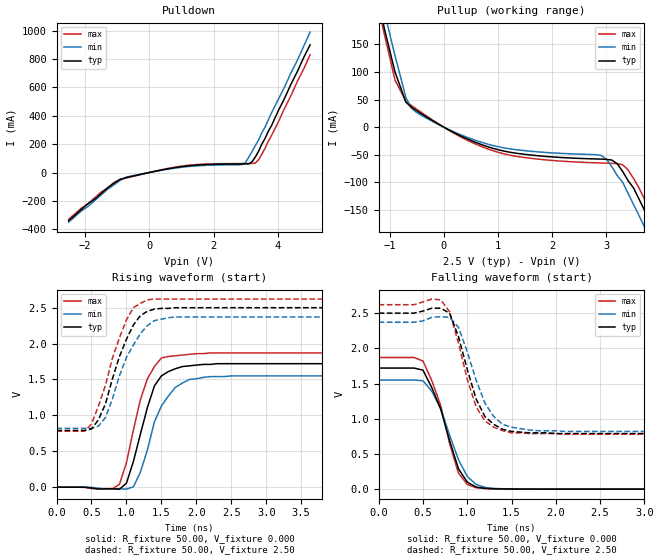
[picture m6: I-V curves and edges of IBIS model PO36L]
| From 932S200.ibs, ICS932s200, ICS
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|   Model PO36L
[Model]   PO36L
Model_type   Output
Polarity   Non-Inverting
Vmeas =   1.25V
Cref =  20.00pF
Rref =  0.000
Vref =   1.25V
C_comp   5.50pF   5.00pF   6.00pF
[Temperature Range]   27.00   70.00   0.000
[Voltage Range]   2.50V   2.37V   2.62V
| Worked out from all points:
|   slope of the pulldown table from 0 to 0.375 V, typ, clamps not added: 21.3 ohm
|   slope of the pullup table from 0 to 0.375 V, typ, clamps not added: 20 ohm
|   rising waveform, R_fixture 50.00, V_fixture 0.000: 20-80 % time 294ps typ, 346ps min, 288ps max; typ from 0 V to 1.72 V
|   rising waveform, R_fixture 50.00, V_fixture 2.50: 20-80 % time 362ps typ, 388ps min, 363ps max; typ from 0.79 V to 2.5 V
|   falling waveform, R_fixture 50.00, V_fixture 0.000: 20-80 % time 265ps typ, 286ps min, 253ps max; typ from 1.72 V to 0 V
|   falling waveform, R_fixture 50.00, V_fixture 2.50: 20-80 % time 257ps typ, 279ps min, 250ps max; typ from 2.5 V to 0.79 V
[Pulldown]
| voltage   I(typ)   I(min)   I(max)
-2.5V     -340mA     -350mA     -330mA
-1.1V     -77.43mA   -88.38mA   -71.31mA
-900mV    -48.05mA   -55.1mA    -48.31mA
-700mV    -34.95mA   -32mA      -37.73mA
1.2V      46.86mA    41.63mA    50.55mA
2.8V      59.88mA    54.77mA    63.39mA
3V        60.16mA    72.42mA    63.65mA
3.2V      77.46mA    150mA      63.96mA
3.3V      110mA      190mA      66.85mA
3.4V      150mA      230mA      89.84mA
4V        430mA      510mA      350mA
5V        900mA      990mA      830mA
[Pullup]
| voltage   I(typ)   I(min)   I(max)
-2.5V     840mA      870mA      820mA
-1.3V     280mA      310mA      260mA
-1.1V     180mA      210mA      170mA
-900mV    100mA      130mA      85.37mA
-700mV    45.28mA    53.96mA    47.05mA
-500mV    29.74mA    26.41mA    32.56mA
1V        -40.82mA   -35.41mA   -45.46mA
2.9V      -57.87mA   -51.13mA   -64.86mA
3.3V      -80.32mA   -100mA     -68.18mA
3.7V      -150mA     -180mA     -130mA
4V        -210mA     -230mA     -180mA
5V        -400mA     -430mA     -380mA
[Ramp]
| variable   typ   min   max
dV/dt_r   1.10/0.30n   1.00/0.34n   1.19/0.27n
dV/dt_f   1.09/0.25n   1.00/0.26n   1.17/0.24n
R_load = 60.00
[Rising Waveform]
R_fixture = 50.00
V_fixture = 0.000
V_fixture_min = 0.000
V_fixture_max = 0.000
| time   V(typ)   V(min)   V(max)
0s        0V         0V         0V
900ps     -27.59mV   -22.59mV   39.23mV
1ns       55.06mV    -26.98mV   340mV
1.1ns     360mV      5.64mV     800mV
1.3ns     1.11V      520mV      1.51V
1.4ns     1.41V      910mV      1.68V
1.5ns     1.55V      1.13V      1.8V
1.7ns     1.65V      1.39V      1.83V
2.1ns     1.71V      1.53V      1.86V
5ns       1.72V      1.55V      1.87V
[Rising Waveform]
R_fixture = 50.00
V_fixture = 2.50
V_fixture_min = 2.37
V_fixture_max = 2.62
| time   V(typ)   V(min)   V(max)
0s        790mV      820mV      780mV
400ps     790mV      820mV      780mV
600ps     940mV      850mV      1.13V
700ps     1.16V      970mV      1.42V
800ps     1.51V      1.23V      1.8V
1ns       2.06V      1.81V      2.33V
1.1ns     2.26V      1.98V      2.5V
1.3ns     2.45V      2.25V      2.61V
1.7ns     2.5V       2.37V      2.62V
5ns       2.5V       2.37V      2.62V
[Falling Waveform]
R_fixture = 50.00
V_fixture = 0.000
V_fixture_min = 0.000
V_fixture_max = 0.000
| time   V(typ)   V(min)   V(max)
0s        1.72V      1.55V      1.87V
500ps     1.69V      1.54V      1.82V
600ps     1.44V      1.39V      1.54V
700ps     1.14V      1.14V      1.19V
800ps     690mV      770mV      650mV
900ps     290mV      420mV      230mV
1ns       100mV      180mV      67.03mV
1.1ns     29.62mV    67.11mV    20.37mV
1.5ns     2.2mV      3.28mV     1.45mV
5ns       2.19uV     -2.53uV    1.35uV
[Falling Waveform]
R_fixture = 50.00
V_fixture = 2.50
V_fixture_min = 2.37
V_fixture_max = 2.62
| time   V(typ)   V(min)   V(max)
0s        2.5V       2.37V      2.62V
700ps     2.57V      2.45V      2.69V
800ps     2.5V       2.44V      2.52V
900ps     2.17V      2.3V       2.08V
1ns       1.7V       1.95V      1.56V
1.1ns     1.28V      1.55V      1.17V
1.2ns     1.03V      1.22V      970mV
1.4ns     850mV      920mV      830mV
2.1ns     790mV      820mV      780mV
5ns       790mV      820mV      780mV
